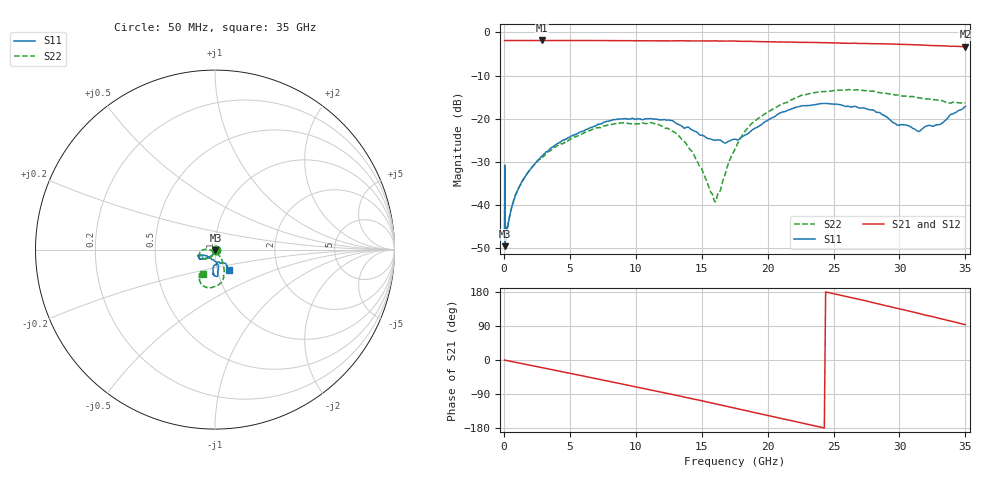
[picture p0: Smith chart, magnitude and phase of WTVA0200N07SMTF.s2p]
! 50 ohm 2-Port S-parameters measured by Modelithics Inc support@modelithics.com  Tampa, FL USA 813-866-6335 (February 2024)
! Smiths Interconnect,  2dB P/N: WTVA0200N07SMTF, Temperature: 25C
! Board: 10 mil Rogers 4350B, Mounting Pad Dimensions: Length: 15 mils, Width: 25 mils, Gap: 40 mils.
# Hz S MA R 50
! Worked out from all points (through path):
!   486 points, 50 MHz to 35 GHz, reference 50 ohm
!   highest |S21| = -1.86 dB at 2.9 GHz (marker M1); lowest = -3.3 dB at 35 GHz (marker M2)
!   group delay of S21, straight-line fit = 21 ps
!   lowest |S11| = -49.6 dB at 90 MHz (marker M3), VSWR 1.01, Z = 50.3 - j0.185 ohm
!   |S11| at or under -10 dB: start of sweep to end of sweep
!   |S22| runs from -49.0 to -13.3 dB; largest |S21 - S12| = 0.018
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5e7  0.005085 -22.1  0.805 -0.4  0.8048 -0.4  0.004096 -13.8
8e7  0.004997 -31.1  0.8058 -0.5  0.8046 -0.6  0.004501 -14.8
9e7  0.003302 -33.8  0.8053 -0.6  0.8052 -0.6  0.003546 -27.8
5e8  0.008291 -79.0  0.8054 -3.4  0.8053 -3.4  0.008414 -77.9
1.1e9  0.01538 -99.2  0.8062 -7.6  0.806 -7.6  0.01564 -96.1
2.9e9  0.03682 -119.0  0.8072 -20.3  0.807 -20.3  0.03619 -114.2
5.9e9  0.07094 -136.9  0.8056 -41.4  0.8056 -41.4  0.06578 -129.1
8.35e9  0.0974 -147.9  0.8033 -59.0  0.8032 -58.9  0.08652 -148.7
1.17e10  0.09753 -160.9  0.7988 -83.3  0.7988 -83.2  0.08535 -169.3
1.39e10  0.07947 -153.2  0.7978 -99.5  0.7975 -99.5  0.04888 177.7
1.49e10  0.06402 -149.9  0.7971 -106.8  0.7972 -106.8  0.02727 -174.1
1.59e10  0.05622 -138.3  0.7977 -114.3  0.798 -114.3  0.01176 -133.7
1.62e10  0.05635 -134.0  0.796 -117.0  0.7963 -116.9  0.01311 -95.7
1.76e10  0.05731 -106.8  0.7944 -127.9  0.7944 -127.7  0.04679 -53.9
1.84e10  0.06534 -88.8  0.788 -133.9  0.788 -133.7  0.07508 -57.3
1.94e10  0.08249 -79.4  0.7825 -141.8  0.7824 -141.5  0.1031 -62.8
2.1e10  0.1173 -81.6  0.776 -153.9  0.7756 -153.7  0.1447 -69.3
2.34e10  0.1437 -83.7  0.7661 -172.5  0.7663 -172.1  0.1982 -84.6
2.74e10  0.1314 -94.7  0.7448 156.5  0.7442 156.6  0.2117 -108.5
2.92e10  0.09893 -95.1  0.7355 141.5  0.7355 142.1  0.1934 -116.4
3.15e10  0.07102 -75.7  0.7152 122.7  0.715 123.3  0.1737 -120.0
3.5e10  0.1389 -55.2  0.6829 93.0  0.6824 93.4  0.1513 -116.5
